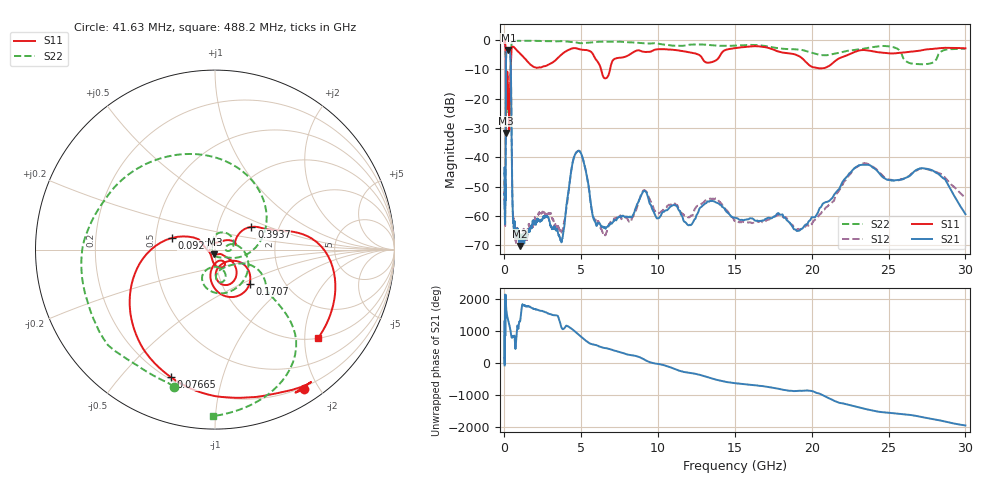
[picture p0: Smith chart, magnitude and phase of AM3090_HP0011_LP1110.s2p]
! Date/Time: Thu, Feb 28, 2019 1:57 PM
! Network Analyzer: Agilent Technologies E8364B Rev: A.07.50.67
! Sweep from 0.010 to 30.000 GHz, 1601 Points, Sweep Type: LOG
! Power Supply: 5.023 V, 0.002 A
# Hz S DB R 50
!freq MagS11 AngS11 MagS21 AngS21 MagS12 AngS12 MagS22 AngS22
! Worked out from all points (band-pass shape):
!   1601 points, 10 MHz to 30 GHz, reference 50 ohm
!   highest |S21| = -3.44 dB at 254.7 MHz (marker M1); lowest = -70.2 dB at 983.6 MHz (marker M2)
!   |S21| within 3 dB of the highest: 104.3 MHz to 396.7 MHz (292.4 MHz wide, 117 % of centre)
!   lowest |S11| = -31.7 dB at 100.9 MHz (marker M3), VSWR 1.05, Z = 49.6 - j2.57 ohm
!   |S11| at or under -10 dB: 91.57 MHz to 409.3 MHz (317.7 MHz wide, 127 % of centre); 6.288 GHz to 6.877 GHz (588.7 MHz wide, 8.94 % of centre)
!   |S22| runs from -33.9 to -0.2 dB; largest |S21 - S12| = 0.01
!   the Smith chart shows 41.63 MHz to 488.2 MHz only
!   S11 on the Smith chart (normalised r, x): 41.63 MHz: 0.17, -1.81; 76.65 MHz: 0.21, -0.69; 92.7 MHz: 0.61, +0.08; 170.7 MHz: 1.35, -0.55; 393.7 MHz: 1.45, +0.39; 488.2 MHz: 1.01, -2.33
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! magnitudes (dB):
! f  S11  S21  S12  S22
! 10 MHz  -0.3  -45.5  -50.3  -0.7
! 38.04 MHz  -0.5  -61.2  -61.3  -1.7
! 41.63 MHz  -0.7  -60.4  -63.2  -2.0
! 76.65 MHz  -2.5  -48.0  -48.8  -4.5
! 92.7 MHz  -12.1  -14.9  -14.9  -12.8
! 100.9 MHz  -31.7  -7.5  -7.5  -33.7
! 144.7 MHz  -19.8  -3.7  -3.7  -24.1
! 170.7 MHz  -11.4  -3.6  -3.5  -14.2
! 254.7 MHz  -22.2  -3.4  -3.4  -17.7
! 312.7 MHz  -30.8  -3.8  -3.8  -16.1
! 393.7 MHz  -12.4  -6.2  -6.2  -10.3
! 488.2 MHz  -2.4  -44.8  -44.3  -0.7
! 550.5 MHz  -2.3  -60.4  -59.9  -0.4
! 983.6 MHz  -4.5  -70.2  -69.6  -0.3
! 2.084 GHz  -9.5  -61.6  -61.0  -0.3
! 3.704 GHz  -5.0  -69.0  -65.5  -0.4
! 4.805 GHz  -3.1  -37.9  -37.7  -1.0
! 5.959 GHz  -6.7  -62.9  -61.7  -0.7
! 7.926 GHz  -5.6  -60.2  -60.6  -0.8
! 19.41 GHz  -6.4  -64.2  -64.5  -3.5
! 23.36 GHz  -3.4  -42.5  -42.0  -3.0
! 30 GHz  -2.9  -59.4  -53.6  -3.0
